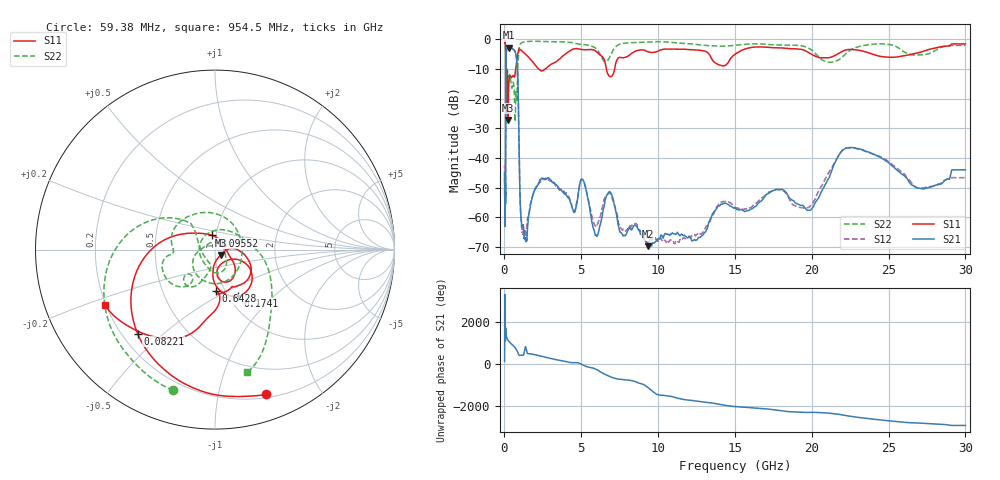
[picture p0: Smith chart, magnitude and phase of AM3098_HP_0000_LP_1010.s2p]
! Date/Time: Thu, Feb 28, 2019 8:31 AM
! Network Analyzer: Agilent Technologies E8364B Rev: A.07.50.67
! Sweep from 0.010 to 30.000 GHz, 1601 Points, Sweep Type: LOG
! Power Supply: 5.023 V, 0.002 A
# Hz S DB R 50
!freq MagS11 AngS11 MagS21 AngS21 MagS12 AngS12 MagS22 AngS22
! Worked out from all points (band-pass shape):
!   1601 points, 10 MHz to 30 GHz, reference 50 ohm
!   highest |S21| = -2.79 dB at 267.8 MHz (marker M1); lowest = -69.7 dB at 9.349 GHz (marker M2)
!   |S21| within 3 dB of the highest: 104.5 MHz to 772.3 MHz (667.8 MHz wide, 152 % of centre)
!   lowest |S11| = -27.2 dB at 232.8 MHz (marker M3), VSWR 1.09, Z = 53.1 - j3.25 ohm
!   |S11| at or under -10 dB: 90.39 MHz to 730.5 MHz (640.1 MHz wide, 156 % of centre); 2.222 GHz to 2.651 GHz (429.3 MHz wide, 17.6 % of centre); 6.633 GHz to 7.168 GHz (535.3 MHz wide, 7.76 % of centre)
!   |S22| runs from -27.6 to -0.6 dB; largest |S21 - S12| = 0.011
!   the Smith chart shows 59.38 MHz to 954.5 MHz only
!   S11 on the Smith chart (normalised r, x): 59.38 MHz: 0.23, -1.39; 82.21 MHz: 0.26, -0.41; 95.52 MHz: 0.96, +0.15; 174.1 MHz: 1.11, -0.63; 642.8 MHz: 0.91, -0.45; 954.5 MHz: 0.20, -0.23
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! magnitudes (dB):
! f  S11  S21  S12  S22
! 10 MHz  -0.3  -47.9  -43.7  -0.6
! 38.04 MHz  -0.5  -61.3  -61.2  -1.0
! 59.38 MHz  -1.4  -48.4  -53.8  -1.7
! 72.54 MHz  -2.2  -54.4  -49.1  -2.6
! 82.21 MHz  -3.9  -31.9  -31.9  -4.4
! 95.52 MHz  -21.9  -9.4  -9.4  -22.9
! 144.7 MHz  -14.4  -3.4  -3.4  -12.7
! 174.1 MHz  -10.8  -3.3  -3.3  -10.0
! 232.8 MHz  -27.2  -2.9  -2.8  -12.4
! 267.8 MHz  -17.1  -2.8  -2.8  -12.7
! 550.5 MHz  -12.2  -3.3  -3.2  -14.5
! 642.8 MHz  -12.7  -3.6  -3.6  -18.8
! 842.3 MHz  -5.6  -9.8  -9.8  -13.6
! 954.5 MHz  -3.3  -37.4  -37.3  -3.0
! 1.076 GHz  -3.6  -60.2  -60.5  -1.3
! 1.335 GHz  -4.9  -67.4  -65.2  -0.8
! 2.084 GHz  -9.2  -49.7  -49.6  -0.6
! 7.926 GHz  -5.9  -65.8  -64.4  -1.2
! 9.349 GHz  -4.2  -69.7  -68.4  -0.9
! 19.7 GHz  -4.2  -57.6  -56.7  -2.7
! 22.67 GHz  -3.4  -36.5  -36.6  -3.2
! 30 GHz  -1.5  -44.0  -46.6  -2.0
